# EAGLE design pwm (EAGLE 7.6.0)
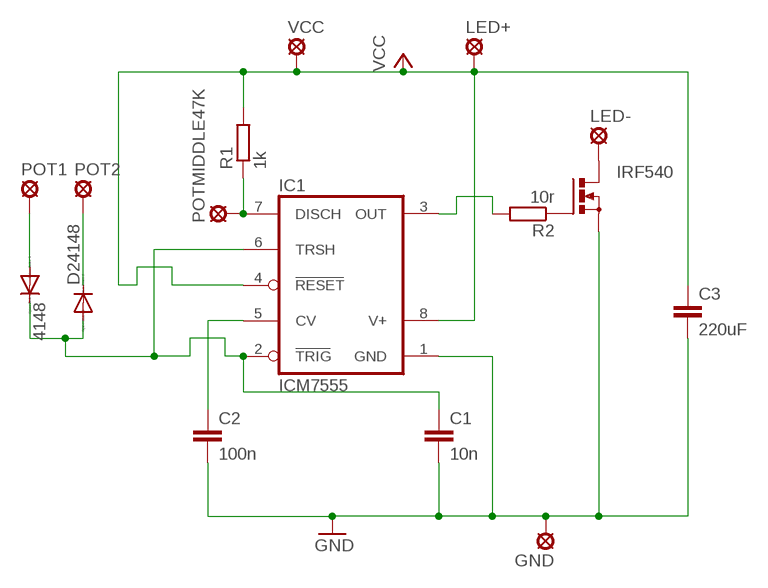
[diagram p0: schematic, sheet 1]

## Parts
4148  1N4148DO35-7  [DO35-7]
C1  10n  C2.5/2  [C2.5-2]
C2  100n  C2.5/2  [C2.5-2]
C3  220uF  C-EU025-060X050  [C025-060X050]
D24148  1N4148DO35-7  [DO35-7]
GND  LSP11  [LSP11]
IC1  ICM7555  [DIL08]
IRF540  PMOSFET_NTO220BV  [TO220BV]
LED+  LSP11  [LSP11]
LED-  LSP11  [LSP11]
POT1  LSP11  [LSP11]
POT2  LSP11  [LSP11]
POTMIDDLE47K  LSP11  [LSP11]
R1  1k  R-EU_0204/7  [0204/7]
R2  10r  R-EU_0204/7  [0204/7]
VCC  LSP11  [LSP11]

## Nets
GND: C1.2 C2.2 C3.2 GND.MP IC1.1(GND) IRF540.S
N$2: IC1.7(DISCH) POTMIDDLE47K.MP R1.1
N$3: C2.1 IC1.5(CV)
N$4: IRF540.D LED-.MP
N$5: 4148.A POT1.MP
N$6: 4148.C C1.1 D24148.A IC1.2(TRIG) IC1.6(TRSH)
N$7: D24148.C POT2.MP
N$8: IC1.3(OUT) R2.2
N$9: IRF540.G R2.1
VCC: C3.1 IC1.4(RESET) IC1.8(V+) LED+.MP R1.2 VCC.MP

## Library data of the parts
4148 D24148 = diode:1N4148: DIODE
C1 C2 = capacitor-wima:C: CAPACITOR
C3 = rcl:C-EU: CAPACITOR, European symbol
GND LED+ LED- POT1 POT2 POTMIDDLE47K VCC = solpad:LSP11: SOLDER PAD
IC1 = maxim:ICM7555: TIMER; MF: MAXIM; MPN: ICM7555IPA+; OC_FARNELL: 9663762; OC_NEWARK: 68K4387
IRF540 = transistor-power:PMOSFET_N: Power MOSFET N-Channel
R1 R2 = resistor:R-EU_: RESISTOR, European symbol

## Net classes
0 default: clearance 0.381 mm

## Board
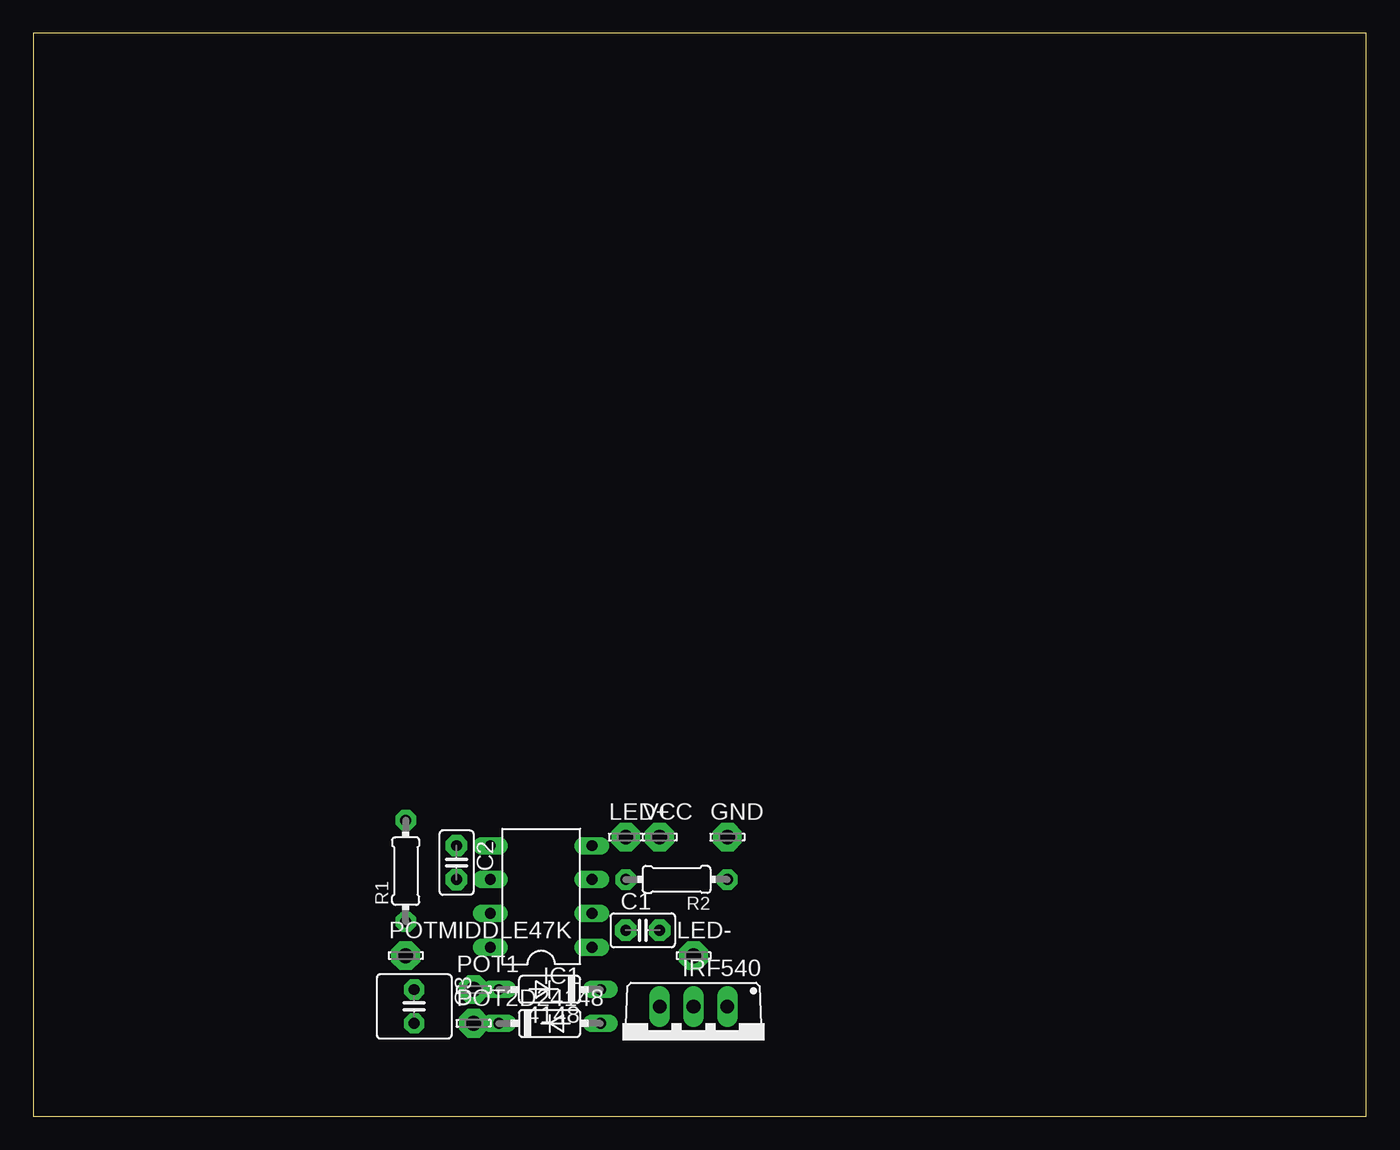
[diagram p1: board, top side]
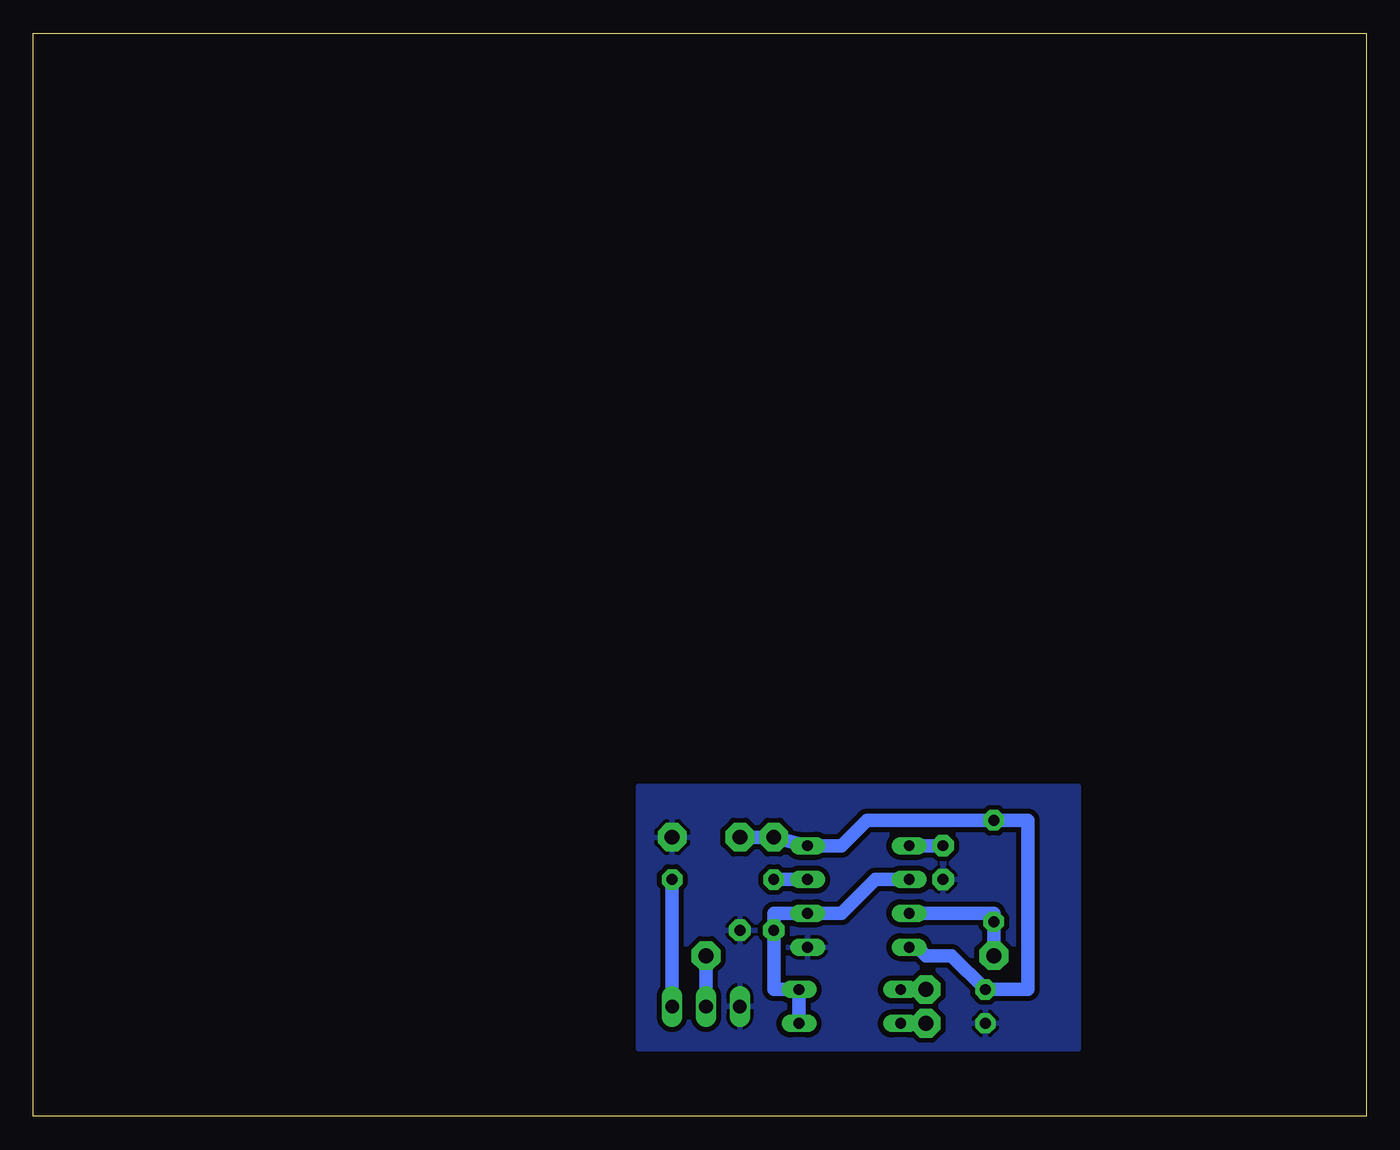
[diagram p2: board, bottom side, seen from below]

Size 100 x 81.27 mm. Coordinates in mm from the lower left corner, seen from the top.
Outline: 0,0 100,0 100,81.27 0,81.27 0,0
Copper layers (1*16): Top 0.035mm / dielectric 1.5mm / Bottom 0.035mm
Design rules "default": minimum track width 10mil, minimum drill 24mil, track to track 8mil, track to pad 8mil, pad to pad 8mil, via to via 8mil, smd to smd 8mil, copper to edge 40mil, drill to drill 8mil, minimum pad ring 10mil, minimum via ring 8mil, stop-mask expansion 4mil, vias tented up to drill 0mil, thermal gap 10mil

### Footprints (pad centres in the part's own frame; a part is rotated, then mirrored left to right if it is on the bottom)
DO35-7 = drill 0.813 long: A 3.81,0; C -3.81,0
C2.5-2 = drill 0.813 pad 1.6 octagon: 1 -1.27,0; 2 1.27,0
C025-060X050 = drill 0.813 pad 1.524 octagon: 1 -1.27,0; 2 1.27,0
LSP11 = drill 1.118 pad 2.159 octagon: MP 0,0
DIL08 = drill 0.813 long: 1 -3.81,-3.81; 2 -1.27,-3.81; 3 1.27,-3.81; 4 3.81,-3.81; 5 3.81,3.81; 6 1.27,3.81; 7 -1.27,3.81; 8 -3.81,3.81
TO220BV = drill 1.016 long: D 0,-2.54; G -2.54,-2.54; S 2.54,-2.54
0204/7 = drill 0.813 pad 1.524 octagon: 1 -3.81,0; 2 3.81,0

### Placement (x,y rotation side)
4148  38.73,9.53 180 top
C1  45.72,13.97 0 top
C2  31.75,19.05 270 top
C3  28.57,8.26 270 top
D24148  38.73,6.98 0 top
GND  52.07,20.95 0 top
IC1  38.1,16.51 90 top
IRF540  49.53,5.71 180 top
LED+  44.45,20.95 0 top
LED-  49.53,12.06 0 top
POT1  33.02,9.53 0 top
POT2  33.02,6.98 0 top
POTMIDDLE47K  27.94,12.06 0 top
R1  27.94,18.41 90 top
R2  48.26,17.78 180 top
VCC  46.99,20.95 0 top

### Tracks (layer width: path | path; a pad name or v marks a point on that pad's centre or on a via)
GND
  pour Bottom: 21.59,24.77 21.59,5.08 54.61,5.08 54.61,24.77
N$2
  Bottom 1.016: POTMIDDLE47K.MP R1.1 27.94,15.24 IC1.7
N$3
  Bottom 1.016: IC1.5 C2.1
N$4
  Bottom 1.016: LED-.MP IRF540.D
N$5
  Bottom 1.016: 4148.A POT1.MP
N$6
  Bottom 1.016: D24148.A 4148.C 44.45,9.53 C1.1 44.45,15.24 IC1.2 39.37,15.24 36.83,17.78 IC1.6
N$7
  Bottom 1.016: D24148.C POT2.MP
N$8
  Bottom 1.016: R2.2 IC1.3
N$9
  Bottom 1.016: R2.1 IRF540.G
VCC
  Bottom 1.016: VCC.MP LED+.MP IC1.4 39.37,20.32 37.47,22.22 R1.2 25.4,22.22 25.4,9.53 C3.1 31.11,12.06 33.02,12.06 33.66,12.7 IC1.8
